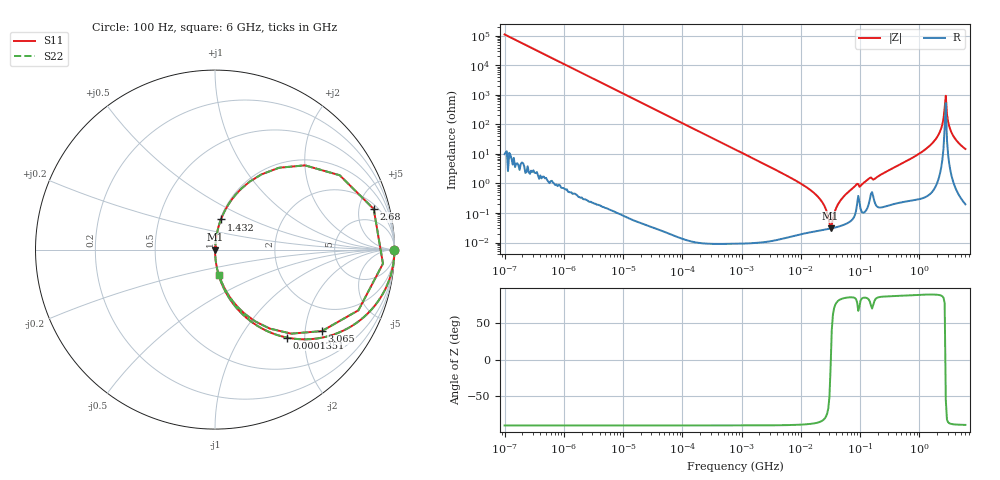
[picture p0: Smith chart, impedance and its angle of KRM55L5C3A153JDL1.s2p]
!Murata Part Number: KRM55L5C3A153JDL1
!These Parameters are Measured in Series Mode Connection
!Data Generated on Jan 08, 2026
!  o--ll--o
!Port1  Port2
!  o------o
!Operation Temp=25[degC], DC Bias Voltage=0[V]
!Freq. Start=100[Hz] Stop=6[GHz] 401[Steps]
# Hz S RI R 50
!Freq.(Hz) S11(Real) S11(Imag) S21(Real) S21(Imag) S12(Real) S12(Imag) S22(Real) S22(Imag)
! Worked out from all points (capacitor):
!   401 points, 100 Hz to 6 GHz, reference 50 ohm
!   read as one part in series: C = 14.4 nF near 109 Hz
!   lowest |Z| = 30.3 mohm at 31.85 MHz (marker M1)
!   series resonance near 32.09 MHz, so ESL is about 1.7 nH
!   S11 on the Smith chart (normalised r, x): 100 Hz: open; 135.1 kHz: 1.00, -1.64; 1.432 GHz: 1.01, +0.35; 2.68 GHz: 2.58, +7.00; 3.065 GHz: 1.19, -2.46; 6 GHz: 1.00, -0.29
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100  1 -0.000905  9e-07 0.000905  9e-07 0.000905  1 -0.000905
2008  0.9997 -0.0182  0.000331 0.0182  0.000331 0.0182  0.9997 -0.0182
11514  0.9893 -0.1031  0.0107 0.1031  0.0107 0.1031  0.9893 -0.1031
40335  0.8824 -0.3221  0.1176 0.3221  0.1176 0.3221  0.8824 -0.3221
135116  0.4008 -0.49  0.5992 0.49  0.5992 0.49  0.4008 -0.49
289253  0.1274 -0.3333  0.8726 0.3333  0.8726 0.3333  0.1274 -0.3333
774597  0.02 -0.1397  0.98 0.1397  0.98 0.1397  0.02 -0.1397
1.555665e7  0.000258 -0.00539  0.9997 0.00539  0.9997 0.00539  0.000258 -0.00539
2.327686e7  0.000269 -0.00223  0.9997 0.00223  0.9997 0.00223  0.000269 -0.00223
3.184506e7  0.000298 -5.16e-05  0.9997 5.16e-05  0.9997 5.16e-05  0.000298 -5.16e-05
3.482834e7  0.000311 0.000561  0.9997 -0.000561  0.9997 -0.000561  0.000311 0.000561
4.556224e7  0.000364 0.00245  0.9996 -0.00245  0.9996 -0.00245  0.000364 0.00245
8.154455e7  0.000896 0.00795  0.9991 -0.00795  0.9991 -0.00795  0.000896 0.00795
3.124326e8  0.00263 0.0283  0.9974 -0.0283  0.9974 -0.0283  0.00263 0.0283
1.431855e9  0.0331 0.1679  0.9669 -0.1679  0.9669 -0.1679  0.0331 0.1679
2.048624e9  0.1473 0.34  0.8527 -0.34  0.8527 -0.34  0.1473 0.34
2.450438e9  0.5011 0.4694  0.4989 -0.4694  0.4989 -0.4694  0.5011 0.4694
2.679998e9  0.8842 0.2264  0.1158 -0.2264  0.1158 -0.2264  0.8842 0.2264
3.065283e9  0.5954 -0.454  0.4046 0.454  0.4046 0.454  0.5954 -0.454
3.352442e9  0.3047 -0.44  0.6953 0.44  0.6953 0.44  0.3047 -0.44
3.8344e9  0.131 -0.3247  0.869 0.3247  0.869 0.3247  0.131 -0.3247
6e9  0.023 -0.1432  0.977 0.1432  0.977 0.1432  0.023 -0.1432
